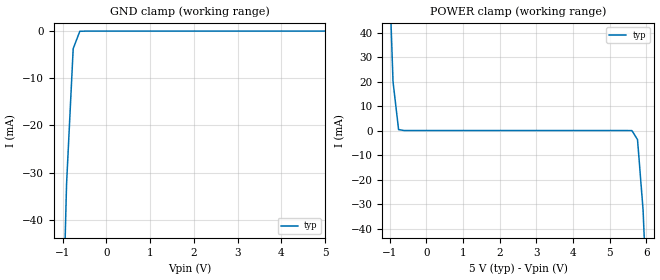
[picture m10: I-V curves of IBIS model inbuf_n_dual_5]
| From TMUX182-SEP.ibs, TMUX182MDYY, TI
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| inbuf_n_dual_5
[Model]   inbuf_n_dual_5
Model_type   Input
Vinl = 0.8
Vinh = 1.35
|   typ   min   max
C_comp   1.598234e-12   NA   NA
[Voltage Range]   5   NA   NA
[Temperature Range]   27   NA   NA
[Power Clamp Reference]   5   NA   NA
[GND Clamp Reference]   0   NA   NA
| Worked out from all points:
|   GND clamp passes 1 mA (typ) near -0.65 V on its own axis
|   POWER clamp passes 1 mA (typ) near -0.76 V on its own axis
[GND Clamp]
|   Voltage   I(typ)   I(min)   I(max)
-10V      -6.183A    NA         NA
-1.061V   -86.95mA   NA         NA
-909.1mV  -32.43mA   NA         NA
-757.6mV  -3.722mA   NA         NA
-606.1mV  -41.78uA   NA         NA
5V        66.34nA    NA         NA
[POWER Clamp]
|   Voltage   I(typ)   I(min)   I(max)
-5V       3.29A      NA         NA
-1.061V   85.94mA    NA         NA
-909.1mV  19.94mA    NA         NA
-757.6mV  393.8uA    NA         NA
-606.1mV  1.601uA    NA         NA
5.606V    -41.78uA   NA         NA
5.758V    -3.722mA   NA         NA
5.909V    -32.43mA   NA         NA
6.061V    -86.95mA   NA         NA
10V       -2.673A    NA         NA
